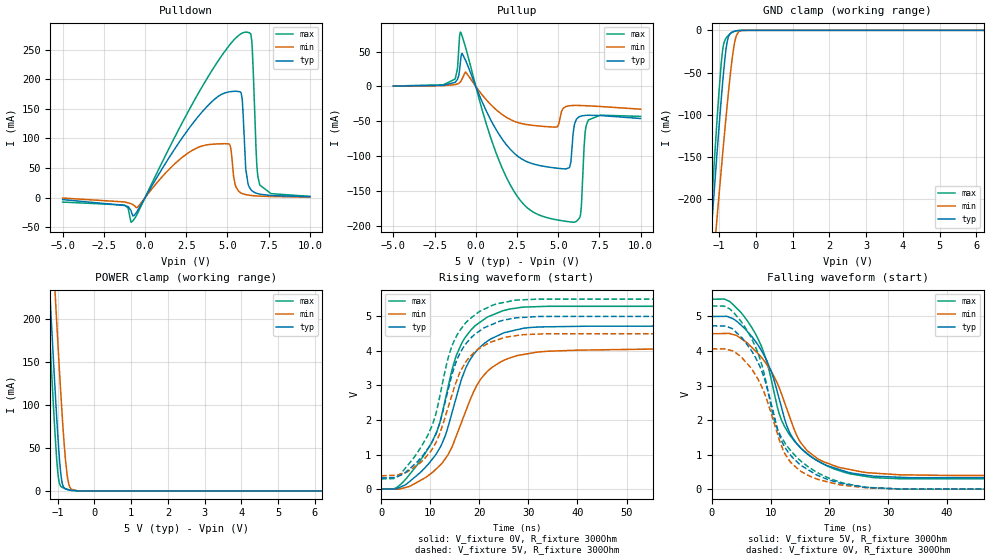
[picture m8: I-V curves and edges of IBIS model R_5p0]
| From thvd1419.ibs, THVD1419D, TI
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|   R_5p0 Model
[Model]   R_5p0
Model_type   3-state
Polarity   Non-Inverting
Vmeas = 2.5
Vref = 0
Cref = 2pF
Rref = 100000
|   typ   min   max
C_comp   4.422pF   4.302pF   4.484pF
| Where Nom  PVT is Nominal Process, 5.0V, 25C
|   Fast PVT is Strong Process,  5.5V, -40C
|   Slow PVT is Weak Process,   4.5V, 150C
[Voltage Range]   5   4.5   5.5
|Junction Temperature
[Temperature Range]   25   150   -40
[Pullup Reference]   5   4.5   5.5
[Pulldown Reference]   0   0   0
[Power Clamp Reference]   5   4.5   5.5
[GND Clamp Reference]   0   0   0
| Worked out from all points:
|   slope of the pulldown table from 0 to 0.75 V, typ, clamps not added: 21 ohm
|   slope of the pullup table from 0 to 0.75 V, typ, clamps not added: 18.5 ohm
|   GND clamp passes 1 mA (typ) near -0.58 V on its own axis
|   POWER clamp passes 1 mA (typ) near -0.67 V on its own axis
|   falling waveform, V_fixture 5V, R_fixture 300Ohm: 20-80 % time 6.49ns typ, 6.69ns min, 6.8ns max; typ from 5 V to 0.323 V
|   rising waveform, V_fixture 0V, R_fixture 300Ohm: 20-80 % time 7.44ns typ, 7.93ns min, 7.42ns max; typ from 0.001 V to 4.73 V
|   rising waveform, V_fixture 5V, R_fixture 300Ohm: 20-80 % time 6.65ns typ, 6.61ns min, 6.85ns max; typ from 0.323 V to 5 V
|   falling waveform, V_fixture 0V, R_fixture 300Ohm: 20-80 % time 6.07ns typ, 5.62ns min, 6.59ns max; typ from 4.73 V to 0.001 V
[Pulldown]
|   Voltage   I(typ)   I(min)   I(max)
-5V       -3.272mA   -664.2uA   -7.474mA
-1.25V    -13.17mA   -7.255mA   -12.42mA
-815mV    -25.38mA   -10.68mA   -41.21mA
2.74V     119.6mA    77.68mA    151.5mA
4.84V     176.7mA    91.08mA    247mA
5.17V     178.8mA    87.21mA    259mA
5.83V     176.7mA    7.735mA    276.7mA
6.1V      52.61mA    5.157mA    279.4mA
6.475V    11.97mA    3.537mA    264.7mA
6.775V    7.308mA    2.84mA     57.1mA
6.97V     5.846mA    2.522mA    21mA
10V       1.556mA    1.006mA    2.167mA
[GND Clamp]
|   Voltage   I(typ)   I(min)   I(max)
-5V       -2.641A    -2.352A    -3.031A
-1.235V   -251mA     -313.8mA   -228mA
-1.13V    -188.2mA   -259.7mA   -155.1mA
-1.07V    -153mA     -229.1mA   -114.9mA
-920mV    -70mA      -154.3mA   -29.31mA
-875mV    -47.91mA   -132.5mA   -16.11mA
-785mV    -14.5mA    -90.57mA   -7.765mA
-725mV    -5.386mA   -64.41mA   -5.068mA
-620mV    -1.606mA   -25.54mA   -1.904mA
-530mV    -550.8uA   -6.168mA   -588.2uA
-365mV    -28.16uA   -188.1uA   -17.2uA
10V       0A         0A         0A
[Pullup]
|   Voltage   I(typ)   I(min)   I(max)
-5V       470.4uA    327uA      589.4uA
-1.25V    5.856mA    2.602mA    10.7mA
-920mV    37.97mA    6.899mA    77.75mA
850mV     -45.44mA   -24.68mA   -69.72mA
2.125V    -91.09mA   -47.86mA   -142.8mA
4.915V    -117.3mA   -58.18mA   -191.5mA
5.77V     -108.2mA   -27.52mA   -194.5mA
5.98V     -54.86mA   -27.32mA   -194.8mA
6.355V    -42.8mA    -27.42mA   -183.9mA
6.625V    -41.62mA   -27.65mA   -67.69mA
6.82V     -41.37mA   -27.86mA   -48.56mA
10V       -46.04mA   -32.66mA   -42.97mA
[POWER Clamp]
|   Voltage   I(typ)   I(min)   I(max)
-5V       3.611A     3.713A     3.566A
-1.415V   403.3mA    518.9mA    349.4mA
-1.25V    263.3mA    379.3mA    208.9mA
-1.175V   201.4mA    317.1mA    147.1mA
-1.07V    118.5mA    232mA      66.29mA
-995mV    64.68mA    173.5mA    21.54mA
-890mV    12.46mA    97.34mA    4.563mA
-815mV    3.162mA    50.92mA    3.03mA
-740mV    1.626mA    18.16mA    1.944mA
-635mV    714.4uA    2.307mA    796.7uA
-455mV    45.03uA    128uA      26.27uA
10V       0A         0A         0A
[Ramp]
R_load = 300
|   typ   min   max
dV/dt_r   2.83718/7.42034e-09   2.4385/7.9003e-09   3.18127/7.39358e-09
dV/dt_f   2.80555/6.47922e-09   2.46916/6.62298e-09   3.12173/6.77209e-09
[Falling Waveform]
V_fixture = 5V
V_fixture_min = 4.5V
V_fixture_max = 5.5V
R_fixture = 300Ohm
C_fixture = 0F
|   Time   V(typ)   V(min)   V(max)
0s        4.999V     4.499V     5.499V
3.156ns   4.965V     4.499V     5.419V
8.025ns   4.129V     3.896V     4.295V
9.485ns   3.663V     3.572V     3.611V
11.47ns   2.604V     2.936V     2.177V
12.7ns    1.859V     2.349V     1.719V
14.04ns   1.414V     1.716V     1.392V
18.38ns   783.1mV    844.9mV    782.1mV
27.43ns   378mV      466.3mV    335.9mV
600ns     323.3mV    384.1mV    296.3mV
[Rising Waveform]
V_fixture = 0V
V_fixture_min = 0V
V_fixture_max = 0V
R_fixture = 300Ohm
C_fixture = 0F
|   Time   V(typ)   V(min)   V(max)
0s        729.5uV    628.9uV    820.8uV
4.471ns   91.23mV    27.33mV    202.5mV
11.09ns   987.1mV    564.7mV    1.58V
13.11ns   1.556V     885.5mV    2.609V
15.22ns   2.601V     1.497V     3.819V
18.24ns   3.765V     2.613V     4.591V
22.11ns   4.324V     3.464V     5.005V
28.85ns   4.65V      3.892V     5.266V
54.32ns   4.715V     4.05V      5.289V
600ns     4.729V     4.065V     5.303V
[Rising Waveform]
V_fixture = 5V
V_fixture_min = 4.5V
V_fixture_max = 5.5V
R_fixture = 300Ohm
C_fixture = 0F
|   Time   V(typ)   V(min)   V(max)
0s        323.3mV    384.1mV    296.3mV
4.138ns   410mV      441.7mV    465.1mV
9.901ns   1.247V     1.054V     1.678V
11.78ns   1.83V      1.545V     2.558V
13.67ns   2.872V     2.368V     3.796V
14.82ns   3.488V     2.896V     4.269V
16.07ns   3.932V     3.385V     4.597V
19.91ns   4.562V     4.064V     5.128V
27.43ns   4.954V     4.439V     5.469V
600ns     4.999V     4.499V     5.499V
[Falling Waveform]
|Gnd
V_fixture = 0V
V_fixture_min = 0V
V_fixture_max = 0V
R_fixture = 300Ohm
C_fixture = 0F
|   Time   V(typ)   V(min)   V(max)
0s        4.729V     4.065V     5.303V
3.008ns   4.68V      4.027V     5.223V
6.454ns   4.078V     3.551V     4.459V
8.901ns   3.225V     2.8V       3.34V
11.01ns   1.844V     1.684V     1.795V
11.99ns   1.353V     1.198V     1.461V
13.49ns   964.4mV    764.4mV    1.097V
18.24ns   381.3mV    274.7mV    452.1mV
26.1ns    54.41mV    44.43mV    54.22mV
600ns     729.5uV    628.9uV    820.8uV
